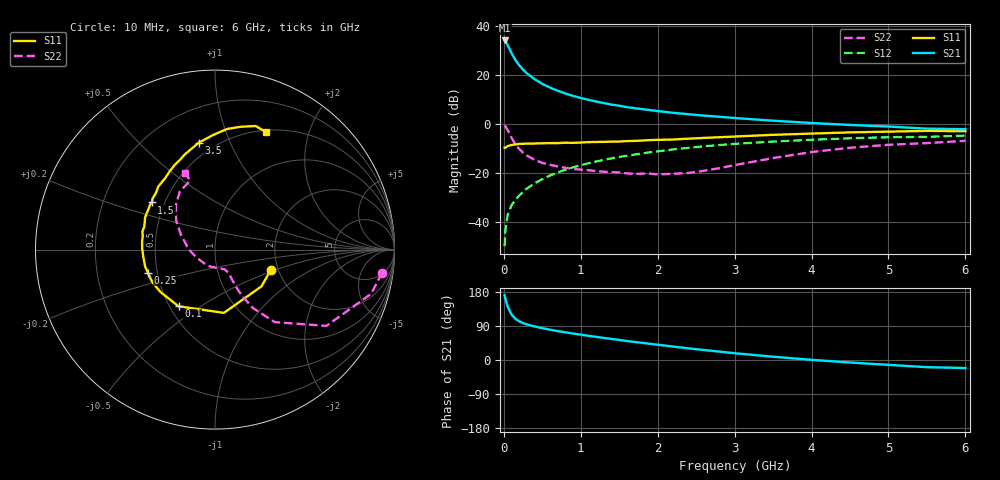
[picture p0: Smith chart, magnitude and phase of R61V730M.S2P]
! SIEMENS Small Signal Semiconductors
! BFR193
! Si NPN RF Bipolar Junction Transistor in SOT23
! VCE = 1.75 V  IC = 30 mA
! Common Emitter S-Parameters:  May  1996
# GHz  S  MA  R  50
!  f  S11  S21  S12  S22
! GHz  MAG  ANG  MAG  ANG  MAG  ANG  MAG  ANG
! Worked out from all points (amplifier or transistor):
!   36 points, 10 MHz to 6 GHz, reference 50 ohm
!   highest |S21| = 33.9 dB at 10 MHz (marker M1)
!   |S21| within 3 dB of that: start of sweep to 67.27 MHz
!   unconditionally stable (mu >= 1): 444.2 MHz to 1.853 GHz
!   at 250 MHz: K = 0.91, MSG = 24.8 dB, |S12| = -27.5 dB
!   at 1.4 GHz: K = 1.02, MAG = 10.0 dB, |S12| = -14.0 dB
!   at 6 GHz: K = 0.96, MSG = 1.3 dB, |S12| = -4.7 dB
!   S11 on the Smith chart (normalised r, x): 10 MHz: 1.82, -0.47; 100 MHz: 0.56, -0.41; 250 MHz: 0.44, -0.13; 1.5 GHz: 0.42, +0.28; 3.5 GHz: 0.41, +0.77; 6 GHz: 0.52, +1.39
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0.01  0.3307 -20.1  49.79 170.8  0.0033 83.1  0.9395 -7.9
0.02  0.3302 -38.4  48.26 161.9  0.0069 79.4  0.9042 -15.8
0.05  0.3559 -82.0  40.17 140.8  0.0142 69.8  0.7524 -34.4
0.1  0.3756 -122.7  27.51 120.1  0.0222 65.9  0.5237 -50.5
0.15  0.3849 -142.1  20.05 108.8  0.029 65.7  0.3885 -57.0
0.2  0.3938 -152.6  15.62 102.1  0.0353 67.7  0.3113 -59.2
0.25  0.3954 -161.1  12.68 97.3  0.042 68.0  0.2615 -60.3
0.3  0.4006 -166.3  10.69 93.9  0.0489 70.3  0.2286 -60.5
0.4  0.4016 -174.7  8.139 88.6  0.0625 71.3  0.1877 -60.3
0.5  0.4056 179.5  6.537 84.0  0.0759 71.6  0.162 -59.8
0.6  0.4088 174.0  5.488 80.0  0.0898 71.3  0.1484 -60.0
0.7  0.4094 169.5  4.742 76.2  0.1038 70.7  0.1379 -61.3
0.8  0.4168 166.0  4.165 73.0  0.1179 69.7  0.1291 -62.9
0.9  0.4143 162.1  3.72 69.8  0.1321 68.9  0.1225 -64.0
1.1  0.4287 155.4  3.101 63.8  0.1594 66.6  0.1153 -69.8
1.5  0.4401 143.3  2.352 53.0  0.2139 61.3  0.1036 -84.4
2.2  0.4844 125.2  1.688 35.5  0.3042 50.9  0.0974 -127.0
3  0.5564 107.6  1.324 17.8  0.3951 38.2  0.1461 179.4
3.5  0.6031 98.5  1.167 8.7  0.4397 30.3  0.2031 157.5
4.5  0.6759 84.2  0.957 -6.6  0.5128 16.1  0.3293 131.5
5.5  0.725 71.8  0.804 -18.9  0.5472 2.1  0.4092 109.7
6  0.7137 66.6  0.784 -21.2  0.5818 -2.0  0.4554 111.2
